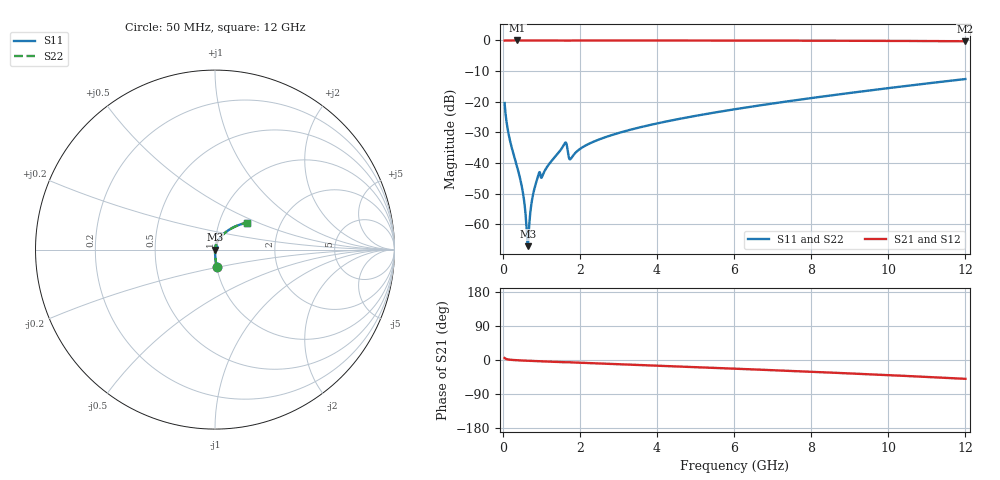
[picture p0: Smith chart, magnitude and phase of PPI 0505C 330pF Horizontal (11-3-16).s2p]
# MHz S MA R 50
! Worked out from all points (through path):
!   1601 points, 50 MHz to 12 GHz, reference 50 ohm
!   highest |S21| = 0.00 dB at 378.6 MHz (marker M1); lowest = -0.3 dB at 12 GHz (marker M2)
!   group delay of S21, straight-line fit = 11.5 ps
!   lowest |S11| = -67.1 dB at 647.5 MHz (marker M3), VSWR 1.00, Z = 50 - j0.0092 ohm
!   |S11| at or under -10 dB: start of sweep to end of sweep
!   |S22| runs from -67.1 to -12.6 dB; largest |S21 - S12| = 0
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50  0.09531 -84.6  0.9953 5.3  0.9953 5.3  0.09531 -84.6
184.4375  0.02404 -88.5  0.9994 0.8  0.9994 0.8  0.02404 -88.5
378.625  0.008485 -88.3  0.9996 -0.7  0.9996 -0.7  0.008485 -88.3
513.0625  0.00363 -85.2  0.9996 -1.4  0.9996 -1.4  0.00363 -85.2
557.875  0.002369 -81.7  0.9996 -1.6  0.9996 -1.6  0.002369 -81.7
610.1562  0.001066 -68.5  0.9995 -1.8  0.9995 -1.8  0.001066 -68.5
647.5  0.000441 -12.0  0.9995 -2.0  0.9995 -2.0  0.000441 -12.0
692.3125  0.001052 62.5  0.9995 -2.2  0.9995 -2.2  0.001052 62.5
744.5938  0.00215 74.9  0.9995 -2.4  0.9995 -2.4  0.00215 74.9
796.875  0.003258 78.4  0.9994 -2.7  0.9994 -2.7  0.003258 78.4
923.8438  0.006351 76.7  0.9988 -3.2  0.9988 -3.2  0.006351 76.7
1043.344  0.006456 77.6  0.9989 -3.6  0.9989 -3.6  0.006456 77.6
1596.031  0.02039 69.5  0.9946 -6.1  0.9946 -6.1  0.02039 69.5
1640.844  0.02148 54.9  0.9893 -6.2  0.9893 -6.2  0.02148 54.9
1767.812  0.01177 65.1  0.996 -6.1  0.996 -6.1  0.01177 65.1
2044.156  0.01768 79.0  0.9986 -7.4  0.9986 -7.4  0.01768 79.0
2791.031  0.02811 78.0  0.9986 -10.3  0.9986 -10.3  0.02811 78.0
4038.312  0.04479 73.7  0.9978 -15.1  0.9978 -15.1  0.04479 73.7
6025  0.07557 66.3  0.9956 -22.9  0.9956 -22.9  0.07557 66.3
8019.156  0.1152 58.2  0.9915 -31.2  0.9915 -31.2  0.1152 58.2
10013.31  0.1672 49.4  0.9837 -40.0  0.9837 -40.0  0.1672 49.4
12000  0.2348 39.9  0.9693 -49.7  0.9693 -49.7  0.2348 39.9
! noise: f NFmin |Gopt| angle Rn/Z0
50  0.0003104  0.8329  0.2478  0.000392
1372  0.003495  0.6367  4.196  0.001811
2701  0.00501  0.5335  8.081  0.001888
4031  0.006479  0.4818  11.78  0.002113
5360  0.007996  0.4548  15.34  0.002419
6682  0.009516  0.4389  18.74  0.002746
8012  0.01109  0.4307  22.01  0.003109
9341  0.01274  0.4287  25.14  0.003521
1.067e+04  0.0145  0.4322  28.16  0.004002
1.2e+04  0.01643  0.4407  31.09  0.004574
